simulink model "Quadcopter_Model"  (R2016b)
settings: Solver=VariableStepAuto  StartTime=0.0  StopTime=10.0  RelTol=1e-3

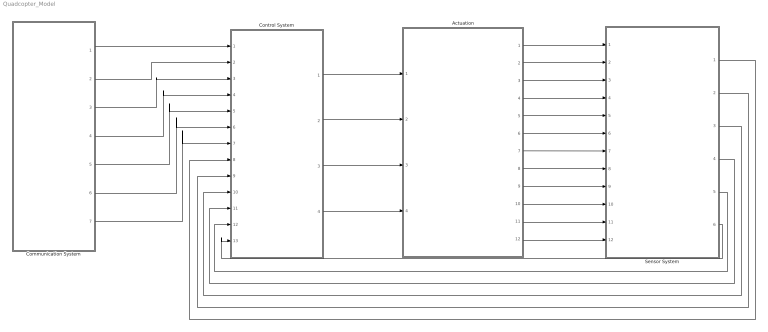
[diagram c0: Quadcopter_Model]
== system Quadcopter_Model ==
  Actuation : Subsystem
  Communication System : Subsystem
  Control System : Subsystem
  Sensor System : Subsystem
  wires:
  Control System/1(Rotor 0 Duty Cycle) -> Actuation/1(Rotor 0 Duty Cycle)
  Control System/2(Rotor 1 Duty Cycle) -> Actuation/2(Rotor 1 Duty Cycle)
  Control System/3(Rotor 2 Duty Cycle) -> Actuation/3(Rotor 2 Duty Cycle)
  Control System/4(Rotor 3 Duty Cycle) -> Actuation/4(Rotor 3 Duty Cycle)
  Actuation/1(Body frame linear velocity (u)) -> Sensor System/1(Body frame linear velocity (u))
  Actuation/2(Body frame linear velocity (v)) -> Sensor System/2(Body frame linear velocity (v))
  Actuation/3(Body frame linear velocity (w)) -> Sensor System/3(Body frame linear velocity (w))
  Actuation/4(Body frame angular velocity (p)) -> Sensor System/4(Body frame angular velocity (p))
  Actuation/5(Body frame angular velocity (q)) -> Sensor System/5(Body frame angular velocity (q))
  Actuation/6(Body frame angular velocity (r)) -> Sensor System/6(Body frame angular velocity (r))
  Actuation/7(Earth frame position (x)) -> Sensor System/7(Earth frame position (x))
  Actuation/8(Earth frame position (y)) -> Sensor System/8(Earth frame position (y))
  Actuation/9(Earth frame position (z)) -> Sensor System/9(Earth frame position (z))
  Actuation/10(Earth frame pitch (phi)) -> Sensor System/10(Earth frame pitch (phi))
  Actuation/11(Earth frame roll (theta)) -> Sensor System/11(Earth frame roll (theta))
  Actuation/12(Earth frame yaw (psi)) -> Sensor System/12(Earth frame yaw (psi))
  Sensor System/6(Yaw rate (psi dot)) -> Control System/13(Yaw rate (psi dot))
  Sensor System/5(Roll rate (theta dot)) -> Control System/12(Roll rate (theta dot))
  Sensor System/4(Pitch rate (phi dot)) -> Control System/11(Pitch rate (phi dot))
  Sensor System/3(Yaw (psi)) -> Control System/10(Yaw (psi))
  Sensor System/2(Roll (theta)) -> Control System/9(Roll (theta))
  Sensor System/1(Pitch (phi)) -> Control System/8(Pitch (phi))
  Communication System/1(x_position) -> Control System/1(x position)
  Communication System/2(y_position) -> Control System/2(y position)
  Communication System/3(z_position) -> Control System/3(z position)
  Communication System/4(x_setpoint) -> Control System/4(x setpoint)
  Communication System/5(y_setpoint) -> Control System/5(y setpoint)
  Communication System/6(z_setpoint) -> Control System/6(z setpoint)
  Communication System/7(yaw_setpoint) -> Control System/7("Yaw setpoint ")

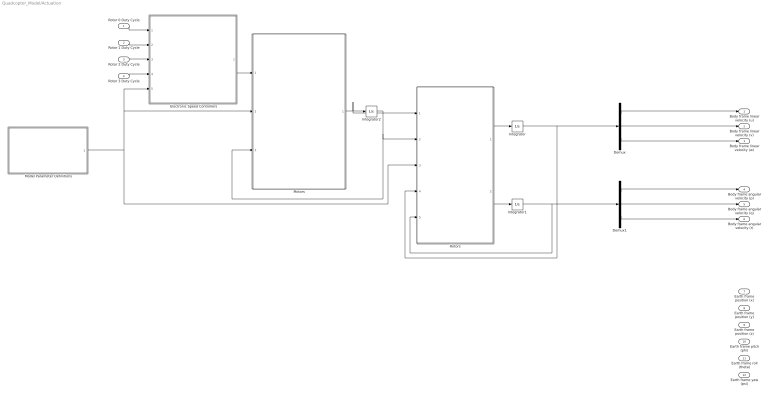
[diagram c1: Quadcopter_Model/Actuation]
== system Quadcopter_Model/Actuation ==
  Rotor 0 Duty Cycle : Inport
  Rotor 1 Duty Cycle : Inport  Port=2
  Rotor 2 Duty Cycle : Inport  Port=3
  Rotor 3 Duty Cycle : Inport  Port=4
  Demux : Demux  Outputs=3
  Demux1 : Demux  Outputs=3
  Electronic Speed Controllers : MATLAB Function  TreatAsAtomicUnit=on
  Integrator : Integrator
  Integrator1 : Integrator
  Integrator2 : Integrator
  Model Parameter Definitions : MATLAB Function  TreatAsAtomicUnit=on
  Motors : MATLAB Function  TreatAsAtomicUnit=on
  Rotors : MATLAB Function  TreatAsAtomicUnit=on
  Body frame linear velocity (u) : Outport
  Body frame linear velocity (v) : Outport  Port=2
  Body frame linear velocity (w) : Outport  Port=3
  Body frame angular velocity (p) : Outport  Port=4
  Body frame angular velocity (q) : Outport  Port=5
  Body frame angular velocity (r) : Outport  Port=6
  Earth frame position (x) : Outport  Port=7
  Earth frame position (y) : Outport  Port=8
  Earth frame position (z) : Outport  Port=9
  Earth frame pitch (phi) : Outport  Port=10
  Earth frame roll (theta) : Outport  Port=11
  Earth frame yaw (psi) : Outport  Port=12
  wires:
  Integrator1/1 -> Rotors/5(bOmega), Demux1/1
  Integrator/1 -> Rotors/4(b_v), Demux/1
  Demux/1 -> Body frame linear velocity (u)/1
  Demux/2 -> Body frame linear velocity (v)/1
  Demux/3 -> Body frame linear velocity (w)/1
  Demux1/1 -> Body frame angular velocity (p)/1
  Demux1/2 -> Body frame angular velocity (q)/1
  Demux1/3 -> Body frame angular velocity (r)/1
  Model Parameter Definitions/1(model_parameters) -> Rotors/3(model_parameters), Electronic Speed Controllers/5(model_parameters), Motors/2(model_parameters)
  Rotor 3 Duty Cycle/1 -> Electronic Speed Controllers/4(rotor_3_duty_cycle)
  Rotor 2 Duty Cycle/1 -> Electronic Speed Controllers/3(rotor_2_duty_cycle)
  Rotor 1 Duty Cycle/1 -> Electronic Speed Controllers/2(rotor_1_duty_cycle)
  Rotor 0 Duty Cycle/1 -> Electronic Speed Controllers/1(rotor_0_duty_cycle)
  Electronic Speed Controllers/1(Vb_eff) -> Motors/1(Vb_eff)
  Motors/1(angular_acceleration) -> Rotors/1(angular_acceleration), Integrator2/1
  Integrator2/1 -> Rotors/2(angular_velocity), Motors/3(angular_velocity)
  Rotors/1(b_v_dot) -> Integrator/1
  Rotors/2(bOmega_dot) -> Integrator1/1

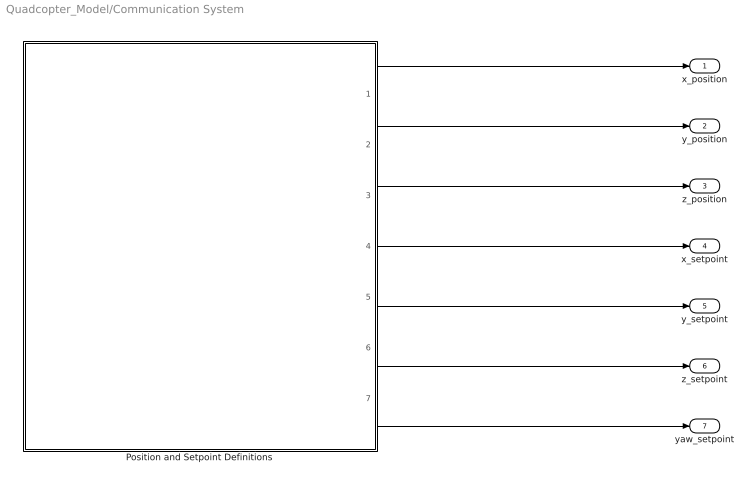
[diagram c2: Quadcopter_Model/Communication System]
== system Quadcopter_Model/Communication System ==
  Position and Setpoint Definitions : MATLAB Function  TreatAsAtomicUnit=on
  x_position : Outport
  y_position : Outport  Port=2
  z_position : Outport  Port=3
  x_setpoint : Outport  Port=4
  y_setpoint : Outport  Port=5
  z_setpoint : Outport  Port=6
  yaw_setpoint : Outport  Port=7
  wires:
  Position and Setpoint Definitions/7(yaw_setpoint) -> yaw_setpoint/1
  Position and Setpoint Definitions/6(z_setpoint) -> z_setpoint/1
  Position and Setpoint Definitions/5(y_setpoint) -> y_setpoint/1
  Position and Setpoint Definitions/4(x_setpoint) -> x_setpoint/1
  Position and Setpoint Definitions/3(z_position) -> z_position/1
  Position and Setpoint Definitions/2(y_position) -> y_position/1
  Position and Setpoint Definitions/1(x_position) -> x_position/1

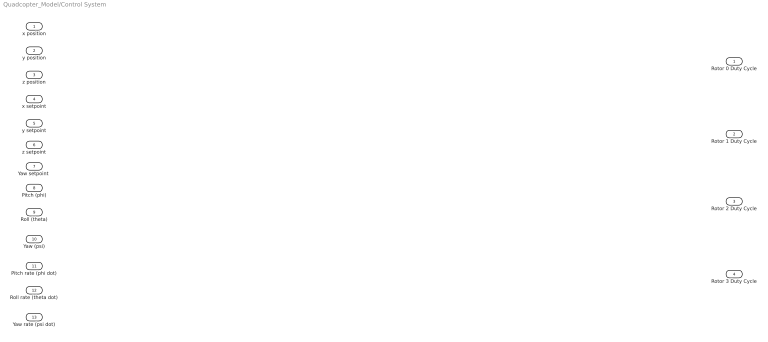
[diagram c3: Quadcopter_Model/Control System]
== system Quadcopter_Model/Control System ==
  x position : Inport
  y position : Inport  Port=2
  z position : Inport  Port=3
  x setpoint : Inport  Port=4
  y setpoint : Inport  Port=5
  z setpoint : Inport  Port=6
  "Yaw setpoint " : Inport  Port=7
  Pitch (phi) : Inport  Port=8
  Roll (theta) : Inport  Port=9
  Yaw (psi) : Inport  Port=10
  Pitch rate (phi dot) : Inport  Port=11
  Roll rate (theta dot) : Inport  Port=12
  Yaw rate (psi dot) : Inport  Port=13
  Rotor 0 Duty Cycle : Outport
  Rotor 1 Duty Cycle : Outport  Port=2
  Rotor 2 Duty Cycle : Outport  Port=3
  Rotor 3 Duty Cycle : Outport  Port=4

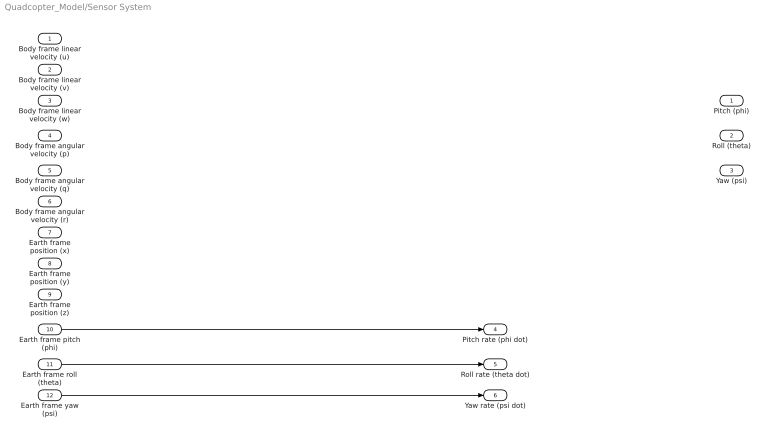
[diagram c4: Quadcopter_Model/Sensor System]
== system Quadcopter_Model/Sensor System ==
  Body frame linear velocity (u) : Inport
  Body frame linear velocity (v) : Inport  Port=2
  Body frame linear velocity (w) : Inport  Port=3
  Body frame angular velocity (p) : Inport  Port=4
  Body frame angular velocity (q) : Inport  Port=5
  Body frame angular velocity (r) : Inport  Port=6
  Earth frame position (x) : Inport  Port=7
  Earth frame position (y) : Inport  Port=8
  Earth frame position (z) : Inport  Port=9
  Earth frame pitch (phi) : Inport  Port=10
  Earth frame roll (theta) : Inport  Port=11
  Earth frame yaw (psi) : Inport  Port=12
  Pitch (phi) : Outport
  Roll (theta) : Outport  Port=2
  Yaw (psi) : Outport  Port=3
  Pitch rate (phi dot) : Outport  Port=4
  Roll rate (theta dot) : Outport  Port=5
  Yaw rate (psi dot) : Outport  Port=6
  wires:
  Earth frame pitch (phi)/1 -> Pitch rate (phi dot)/1
  Earth frame roll (theta)/1 -> Roll rate (theta dot)/1
  Earth frame yaw (psi)/1 -> Yaw rate (psi dot)/1

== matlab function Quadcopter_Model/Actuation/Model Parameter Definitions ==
function model_parameters = modelParameterDefinitions()
%This function defines and returns the quadcopter parameters used, as a
%struct.

    %Create an empty struct
    model_parameters = struct();
    
    %Fill model_parameters struct with the parameters of the quadcopter
    model_parameters.m = 1.19;            % Quadrotor + battery mass
    model_parameters.g = 9.81;            % Acceleration of gravity
    model_parameters.Jxx = 0.0218;        % Quadrotor and battery motor of inertia around bx (pitch)
    model_parameters.Jyy = 0.0277;        % Quadrotor and battery motor of inertia around by (roll)
    model_parameters.Jzz = 0.0332;        % Quadrotor and battery motor of inertia around bz (yaw)
    model_parameters.J = [model_parameters.Jxx, 0 , 0; ... % Quadrotor moment of inertia matrix
                           0, model_parameters.Jyy, 0; ...
                           0,  0, model_parameters.Jzz]; 
    model_parameters.Jreq = 4.2012e-05;   % Rotor and motor moment of inertia around axis of rotation
    model_parameters.Kt = 8.1558*10^-6;   % Rotor thrust constant
    model_parameters.Kh = 0;              % Rotor in-plane drag constant
    model_parameters.Kd = 1.8087e-07;     % Rotor drag constant
    model_parameters.rhx = 0.016;         % X-axis distance from center of mass to a rotor hub
    model_parameters.rhy = 0.016;         % Y-axis distance from center of mass to a rotor hub
    model_parameters.rhz = 0.003;         % Z-axis distance from center of mass to a rotor hub
    model_parameters.Rm = 0.2308;         % Motor resistance
    model_parameters.Kq = 96.3422;        % Motor torque constant
    model_parameters.Kv = 96.3422;        % Motor back emf constant
    model_parameters.If = 0.511;          % Motor internal friction current
    model_parameters.Pmin = 0.47;         % Minimum zybo output duty cycle command
    model_parameters.Pmax = 0.80;         % Maximum zybo output duty cycle command
    model_parameters.Tc = 0.01;           % Camera system sampling period
    model_parameters.tau_c = 0;           % Camera system total latency
    model_parameters.Vb = 11.1;           % Nominal battery voltage (V)
    
end

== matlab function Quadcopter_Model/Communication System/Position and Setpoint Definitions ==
function [x_position, y_position, z_position, x_setpoint,...
    y_setpoint, z_setpoint, yaw_setpoint]= positionAndSetpointDefinitions

x_position = 0;
y_position = 0;
z_position = 0;
x_setpoint = 0;
y_setpoint = 0;
z_setpoint = 0;
yaw_setpoint = 0;

end

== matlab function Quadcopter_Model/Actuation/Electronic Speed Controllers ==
function Vb_eff   = ESC(rotor_0_duty_cycle, rotor_1_duty_cycle, rotor_2_duty_cycle, rotor_3_duty_cycle, model_parameters)

% Pull parameters from the model_parameters struct
Pmin = model_parameters.Pmin;
Pmax = model_parameters.Pmax;
Vb = model_parameters.Vb;

% Define u_Pi for each of the rotors
u_P0 = (rotor_0_duty_cycle/100 - Pmin) / (Pmax - Pmin);
u_P1 = (rotor_1_duty_cycle/100 - Pmin) / (Pmax - Pmin);
u_P2 = (rotor_2_duty_cycle/100 - Pmin) / (Pmax - Pmin);
u_P3 = (rotor_3_duty_cycle/100 - Pmin) / (Pmax - Pmin);

% Determine the effective battery voltage from each ESC
Vb_eff_0 = u_P0 * Vb;
Vb_eff_1 = u_P1 * Vb;
Vb_eff_2 = u_P2 * Vb;
Vb_eff_3 = u_P3 * Vb;

Vb_eff = [Vb_eff_0, Vb_eff_1, Vb_eff_2, Vb_eff_3];

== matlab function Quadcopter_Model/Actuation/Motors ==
function angular_acceleration  = motor(Vb_eff, model_parameters, angular_velocity)

% Pull parameters from the model_parameters struct
Rm = model_parameters.Rm;
Kv = model_parameters.Kv;
Kq = model_parameters.Kq;
Kd = model_parameters.Kd;
If = model_parameters.If;
Jreq = model_parameters.Jreq;

% Define each motors effective battery voltage
Vb_eff_0 = Vb_eff(1);
Vb_eff_1 = Vb_eff(2);
Vb_eff_2 = Vb_eff(3);
Vb_eff_3 = Vb_eff(4);

% Determine the angular velocity of each rotor from feedback
w_0 = angular_velocity(1);
w_1 = angular_velocity(2);
w_2 = angular_velocity(3);
w_3 = angular_velocity(4);

% Determine angular acceleration of each rotor
w_0_dot = 1/(Jreq*Rm*Kq) * Vb_eff_0 - 1/(Jreq*Rm*Kq*Kv) * w_0 - 1/(Jreq*Kq)*If - (Kd/Jreq) * w_0^2;
w_1_dot = 1/(Jreq*Rm*Kq) * Vb_eff_1 - 1/(Jreq*Rm*Kq*Kv) * w_1 - 1/(Jreq*Kq)*If - (Kd/Jreq) * w_1^2;
w_2_dot = 1/(Jreq*Rm*Kq) * Vb_eff_2 - 1/(Jreq*Rm*Kq*Kv) * w_2 - 1/(Jreq*Kq)*If - (Kd/Jreq) * w_2^2;
w_3_dot = 1/(Jreq*Rm*Kq) * Vb_eff_3 - 1/(Jreq*Rm*Kq*Kv) * w_3 - 1/(Jreq*Kq)*If - (Kd/Jreq) * w_3^2;

angular_acceleration = [w_0_dot, w_1_dot, w_2_dot, w_3_dot];

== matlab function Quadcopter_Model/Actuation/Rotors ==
function [b_v_dot, bOmega_dot]= rotor(angular_acceleration, angular_velocity, model_parameters,b_v, bOmega)

% Pull parameters from the model_parameters struct
m = model_parameters.m;
Kd = model_parameters.Kd;
Kt = model_parameters.Kt;
rhx = model_parameters.rhx;
rhy = model_parameters.rhy;
rhz = model_parameters.rhz;
Jreq = model_parameters.Jreq;
J = model_parameters.J;

% Create r_hi vector
rhi = [rhx; rhy; rhz];

% Define vector from body frame origin to center of mass
br_oc = 0;

% Define 3x3 Identity Matrix
I = eye(3);

% Create gamma vectors
gamma_Ti = [0; 0; -1];
gamma_omega_03 = [0; 0; 1];  %Rotors 0 and 3 use this gamma_omega vector
gamma_omega_12 = [0; 0; -1]; %Rotors 1 and 2 use this gamma_omega vector

% Define angular velocities for each rotor
w_0 = angular_velocity(1);
w_1 = angular_velocity(2);
w_2 = angular_velocity(3);
w_3 = angular_velocity(4);

% Define angular acceleration for each rotor
w_0_dot = angular_acceleration(1);
w_1_dot = angular_acceleration(2);
w_2_dot = angular_acceleration(3);
w_3_dot = angular_acceleration(4);

% Define the body force in the z-direction from each rotor
bF_0 = Kt * w_0 * w_0 * gamma_Ti;
bF_1 = Kt * w_1 * w_1 * gamma_Ti;
bF_2 = Kt * w_2 * w_2 * gamma_Ti;
bF_3 = Kt * w_3 * w_3 * gamma_Ti;

% Sum up the body forces in the z-direction from each vector to get the
% total body force in the z-direction
bF = bF_0 + bF_1 + bF_2 + bF_3;


% Define the in-plane drag and induced torque produced by each rotor
bQ_d0 = -1 * Kd * w_0 * w_0 * gamma_omega_03;
bQ_d1 = -1 * Kd * w_1 * w_1 * gamma_omega_12;
bQ_d2 = -1 * Kd * w_2 * w_2 * gamma_omega_12;
bQ_d3 = -1 * Kd * w_3 * w_3 * gamma_omega_03;

% Sum up the total in-plane drag and induced torque to get the total
% in-plane drag and induced torque on the body
bQ_d = bQ_d0 + bQ_d1 + bQ_d2 + bQ_d3;

% Define the force lever arm torque created from the force produced by each
% rotor in the z-direction
bQ_F = cross( rhi, bF );

%Define the change in angular momentum torque produced by each rotor 
bQ_L0 = -1 * Jreq * ( cross(bOmega, w_0 * gamma_omega_03) + w_0_dot * gamma_omega_03 );
bQ_L1 = -1 * Jreq * ( cross(bOmega, w_1 * gamma_omega_12) + w_1_dot * gamma_omega_12 ); 
bQ_L2 = -1 * Jreq * ( cross(bOmega, w_2 * gamma_omega_12) + w_2_dot * gamma_omega_12 ); 
bQ_L3 = -1 * Jreq * ( cross(bOmega, w_3 * gamma_omega_03) + w_3_dot * gamma_omega_03 );

% Sum up the total change in angular momentum torque produced by each rotor
bQ_L = bQ_L0 + bQ_L1 + bQ_L2 + bQ_L3;

% Define the total rotor system torque as the sum of the in-plane drag and
% induced torque, force lever arm torque, and change in angular momentum
% torques
bQ = bQ_d + bQ_F + bQ_L;

% Define the body frame linear velocities
b_v_dot = (m*I)^(-1) * ( bF - cross( bOmega, m*(b_v + cross(bOmega, br_oc)) ) );

% Define the body frame angular velocities
bOmega_dot = J ^(-1) * ( bQ - cross(bOmega, J * bOmega) - cross(br_oc, bF) );
